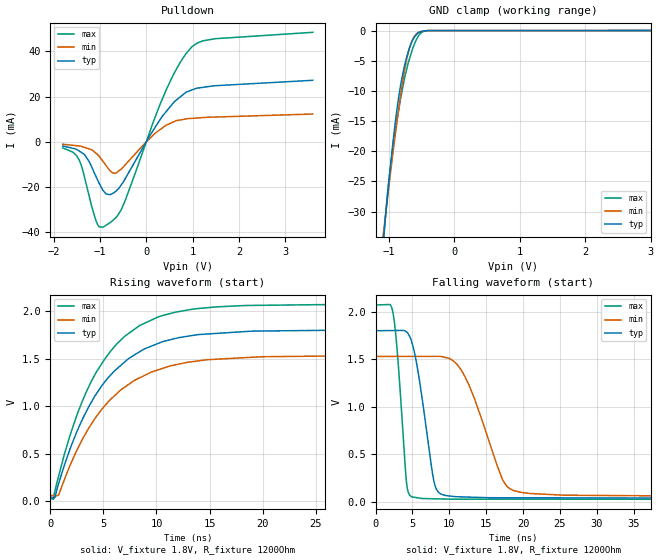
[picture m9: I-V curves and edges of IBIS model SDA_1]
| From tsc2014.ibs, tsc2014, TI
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|   1.8V SDA Model
[Model] SDA_1
Model_type I/O_open_drain
Polarity   Non-Inverting
Enable   Active-Low
Vinl = 0.54
Vinh = 1.26
Vmeas = 0.9
Vref = 0.9
Cref = 15pF
Rref = 50
|   typ   min   max
|   C_comp tri-state
C_comp   3.1256960e-12   3.0017270e-12   3.3008290e-12
|   C_comp high output
|C_comp   2.8228490e-11   2.4306570e-11   2.9676920e-11
|   C_comp low output
|C_comp   3.1256960e-12   3.3008290e-12   3.0017270e-12
|Where nom PVT is NOM Process, 1.8V,27C
|   Fast PVT is Strong Process, 2.07V, -40C
|   Slow PVT is Weak Process, 1.53V, 85C
[Model Spec]
Vinl   0.54   0.459   0.621
Vinh   1.26   1.071   1.449
| VINL 0.3 DVDD, VINH 0.7 DVDD
[Voltage Range]   1.8   1.53   2.07
[Temperature Range]   27   85   -40
[Pullup Reference]   1.8   1.53   2.07
[Pulldown Reference]   0   0   0
[Power Clamp Reference]   1.8   1.53   2.07
[GND Clamp Reference]   0   0   0
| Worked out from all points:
|   slope of the pulldown table from 0 to 0.27 V, typ, clamps not added: 30.3 ohm
|   GND clamp passes 1 mA (typ) near -0.60 V on its own axis
|   falling waveform, V_fixture 1.8V, R_fixture 1200Ohm: 20-80 % time 1.96ns typ, 4.02ns min, 1.11ns max; typ from 1.8 V to 0.041 V
|   rising waveform, V_fixture 1.8V, R_fixture 1200Ohm: 20-80 % time 5.47ns typ, 5.7ns min, 5.14ns max; typ from 0.041 V to 1.8 V
[Pulldown]
|   Voltage   I(typ)   I(min)   I(max)
-1.8V     -1.814mA   -1.046mA   -2.65mA
-1.451V   -3.975mA   -1.817mA   -7.807mA
-1.331V   -5.638mA   -2.431mA   -15.63mA
-1.089V   -15mA      -4.909mA   -34.47mA
-932.5mV  -21.42mA   -8.634mA   -37.65mA
-725.8mV  -22.76mA   -13.65mA   -34.79mA
-547.2mV  -19.26mA   -12.12mA   -30.28mA
431mV     13.37mA    7.357mA    22.93mA
723.5mV   19.65mA    9.628mA    34.75mA
987.2mV   22.9mA     10.37mA    41.97mA
1.489V    24.78mA    10.95mA    45.53mA
3.595V    27.17mA    12.28mA    48.34mA
[GND Clamp]
|   Voltage   I(typ)   I(min)   I(max)
-1.8V     -127mA     -105mA     -167.2mA
-1.077V   -34.16mA   -33.2mA    -34.57mA
-1.068V   -33.1mA    -32.37mA   -33.24mA
-988.6mV  -24.13mA   -25.09mA   -23.94mA
-894.9mV  -14.82mA   -16.86mA   -16.46mA
-813.8mV  -8.792mA   -10.42mA   -11.02mA
-753.4mV  -5.64mA    -6.341mA   -7.687mA
-683.2mV  -2.913mA   -2.924mA   -4.717mA
-618mV    -1.291mA   -1.132mA   -2.54mA
-539.6mV  -330.3uA   -238uA     -815.6uA
-408.8mV  -13.77uA   -9.929uA   -19.64uA
3.595V    0A         0A         0A
[POWER Clamp]
|   SCR cell for ESD function. Effects occurr above VDD x 2
|   Voltage   I(typ)   I(min)   I(max)
-1.8V     0A         0A         0A
0V        0A         0A         0A
3.6V      0A         0A         0A
[Ramp]
R_load = 1200
|   typ   min   max
dV/dt_r   1.05551/5.40895e-009  0.882934/5.65113e-009   1.22477/5.1347e-009
dV/dt_f   1.0555/1.95557e-009  0.882452/3.99913e-009   1.22477/1.10831e-009
[Falling Waveform]
V_fixture = 1.8V
V_fixture_min = 1.53V
V_fixture_max = 2.07V
R_fixture = 1200Ohm
C_fixture = 0F
|   Time   V(typ)   V(min)   V(max)
0s        1.8V       1.53V      2.07V
2.363ns   1.802V     1.53V      1.986V
3.087ns   1.802V     1.53V      1.437V
4.177ns   1.788V     1.53V      216.8mV
4.875ns   1.688V     1.53V      55.63mV
7.871ns   232.4mV    1.53V      34.64mV
8.917ns   81.93mV    1.528V     32.77mV
12.09ns   53.44mV    1.322V     30.55mV
18.65ns   45.07mV    123.1mV    30.23mV
50ns      40.83mV    59.24mV    28.72mV
[Rising Waveform]
V_fixture = 1.8V
V_fixture_min = 1.53V
V_fixture_max = 2.07V
R_fixture = 1200Ohm
C_fixture = 0F
|   Time   V(typ)   V(min)   V(max)
0s        40.81mV    58.43mV    28.72mV
300.1ps   33.44mV    57.05mV    17.8mV
813.3ps   194mV      68.72mV    273.5mV
2.518ns   734.5mV    537.2mV    908.4mV
4.35ns    1.131V     890.4mV    1.361V
6.933ns   1.457V     1.194V     1.728V
10.11ns   1.658V     1.38V      1.936V
13.91ns   1.753V     1.476V     2.027V
19.87ns   1.791V     1.52V      2.061V
50ns      1.8V       1.53V      2.07V
